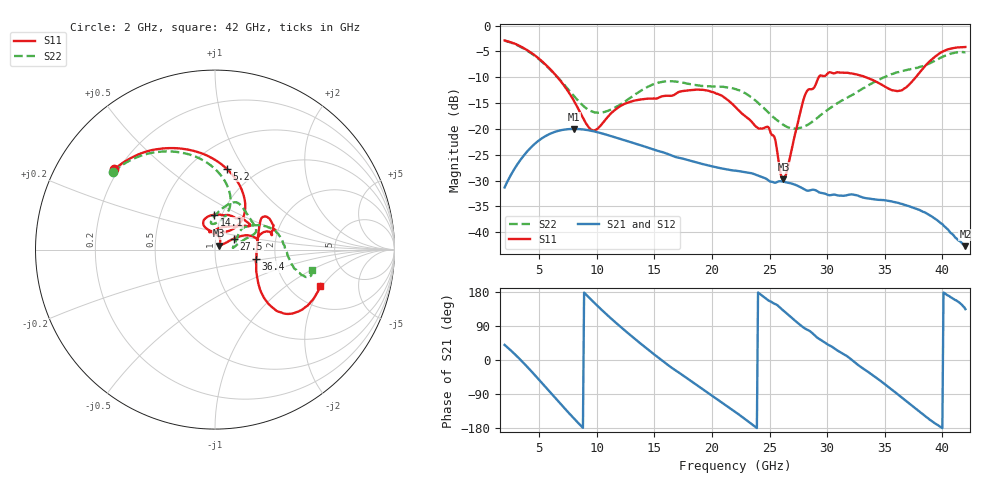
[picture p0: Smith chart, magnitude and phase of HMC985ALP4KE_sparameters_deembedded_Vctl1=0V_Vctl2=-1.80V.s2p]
!s2p File: Measurements: S11, S21, S12, S22
# GHz S dB R 50.0
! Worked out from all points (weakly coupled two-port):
!   401 points, 2 GHz to 42 GHz, reference 50 ohm
!   highest |S21| = -20.00 dB at 8 GHz (marker M1); lowest = -42.7 dB at 42 GHz (marker M2)
!   lowest |S11| = -29.7 dB at 26.2 GHz (marker M3), VSWR 1.07, Z = 52.4 + j2.36 ohm
!   |S11| at or under -10 dB: 6.591 GHz to 29.27 GHz (22.68 GHz wide, 126 % of centre); 33.36 GHz to 37.7 GHz (4.334 GHz wide, 12.2 % of centre)
!   |S22| runs from -20.0 to -2.9 dB; largest |S21 - S12| = 0.00018
!   S11 on the Smith chart (normalised r, x): 2 GHz: 0.18, +0.34; 5.2 GHz: 0.73, +0.84; 14.1 GHz: 0.92, +0.37; 27.5 GHz: 1.22, +0.15; 36.4 GHz: 1.58, -0.18; 42 GHz: 2.90, -1.91
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2  -2.88 141.5  -31.34 39.8  -31.34 39.9  -2.92 142.7
3.6  -4.29 112.2  -25.34 -6.4  -25.35 -6.4  -4.39 115.0
5.2  -6.82 81.9  -21.88 -59.3  -21.89 -59.3  -6.93 90.1
8  -14.49 46.7  -20.00 -153.7  -20.00 -153.7  -13.59 71.5
8.7  -17.44 52.1  -20.09 -175.9  -20.09 -175.9  -15.28 76.9
9.8  -20.30 87.1  -20.50 150.6  -20.51 150.5  -16.80 90.6
12.1  -15.52 113.0  -21.99 86.6  -21.99 86.6  -15.20 94.4
14.1  -14.22 91.1  -23.37 36.1  -23.38 36.1  -12.25 77.5
15.4  -13.94 73.1  -24.32 5.2  -24.32 5.2  -11.02 69.2
19.3  -12.46 34.4  -26.86 -79.3  -26.88 -79.3  -11.68 39.9
22  -15.67 52.3  -28.08 -136.4  -28.09 -136.5  -12.27 22.5
25  -20.11 98.3  -30.14 155.5  -30.14 155.5  -17.06 15.4
26.2  -29.74 43.6  -30.22 130.3  -30.22 130.3  -19.22 8.0
27.5  -18.36 30.0  -31.10 96.5  -31.10 96.4  -19.88 6.8
28.1  -13.33 20.8  -31.80 82.7  -31.80 82.8  -19.45 11.6
28.7  -12.29 12.9  -31.79 71.3  -31.80 71.4  -18.62 17.7
31  -9.06 23.3  -32.91 23.2  -32.91 23.1  -14.87 37.3
33.3  -9.94 34.3  -33.38 -26.2  -33.41 -26.2  -11.95 32.2
35.4  -12.27 12.2  -33.99 -73.2  -33.98 -73.3  -9.60 21.1
36.4  -12.58 -13.0  -34.50 -97.1  -34.51 -97.3  -8.83 14.4
39.5  -5.81 -43.3  -37.59 -170.0  -37.65 -169.9  -6.60 -14.1
42  -4.14 -19.0  -42.71 134.1  -42.75 134.1  -5.15 -11.7
